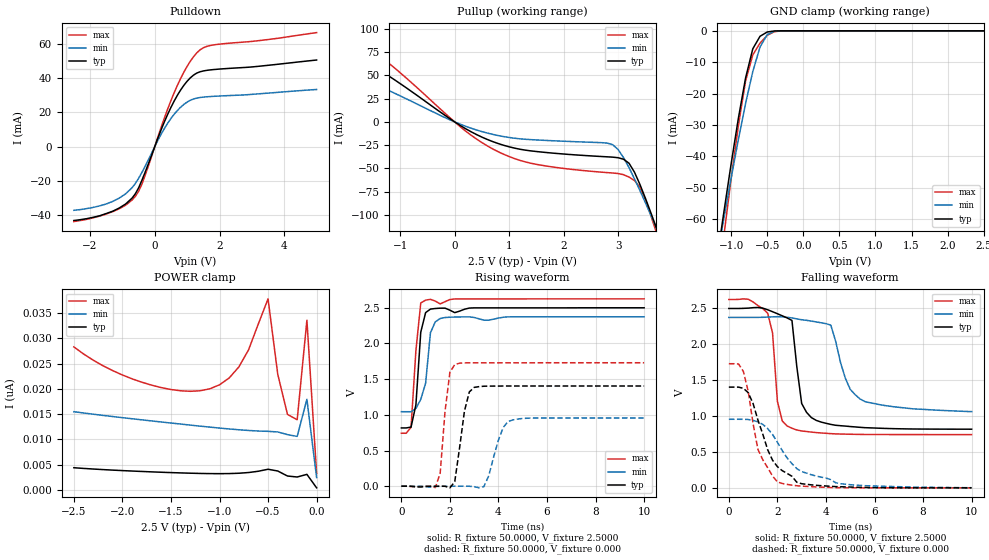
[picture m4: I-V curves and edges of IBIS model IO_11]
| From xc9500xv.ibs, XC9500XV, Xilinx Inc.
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|   Model IO_11
[Model]   IO_11
Model_type   I/O
Polarity   Non-Inverting
Enable   Active-High
Vinl =   0.8000V
Vinh =   2.0000V
Vmeas =   1.2500V
Cref =  35.0000pF
Rref =   1.0000M
Vref =  0.000V
C_comp   1.8820pF   1.2910pF   2.4730pF
[Temperature Range]   25.0000   100.0000   0.000
[Voltage Range]   2.5000V   2.3750V   2.6250V
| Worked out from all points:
|   slope of the pulldown table from 0 to 0.375 V, typ, clamps not added: 21 ohm
|   slope of the pullup table from 0 to 0.375 V, typ, clamps not added: 29.3 ohm
|   GND clamp passes 1 mA (typ) near -0.55 V on its own axis
|   rising waveform, R_fixture 50.0000, V_fixture 2.5000: 20-80 % time 201ps typ, 305ps min, 250ps max; typ from 0.817 V to 2.5 V
|   rising waveform, R_fixture 50.0000, V_fixture 0.000: 20-80 % time 361ps typ, 497ps min, 284ps max; typ from 0 V to 1.4 V
|   falling waveform, R_fixture 50.0000, V_fixture 2.5000: 20-80 % time 383ps typ, 792ps min, 329ps max; typ from 2.5 V to 0.818 V
|   falling waveform, R_fixture 50.0000, V_fixture 0.000: 20-80 % time 1.01ns typ, 1.56ns min, 711ps max; typ from 1.4 V to 0 V
[Pulldown]
| voltage   I(typ)   I(min)   I(max)
-2.5V     -43.3mA    -37.3mA    -43.9mA
-1.9V     -41.4mA    -35.6mA    -41.7mA
-1.3V     -37.85mA   -32.1mA    -38.1mA
-900mV    -33.61mA   -27.65mA   -34.3mA
-600mV    -27.65mA   -21.57mA   -29.14mA
-400mV    -19.86mA   -15.23mA   -22.08mA
200mV     10.04mA    7.385mA    11.51mA
600mV     26.71mA    18.98mA    31.58mA
1V        38.31mA    26.1mA     47.05mA
1.4V      43.85mA    28.77mA    56.7mA
1.8V      45.11mA    29.44mA    59.52mA
5V        50.73mA    33.47mA    66.81mA
[Pullup]
| voltage   I(typ)   I(min)   I(max)
-2.5V     70.1mA     45.22mA    94.12mA
-2.3V     77.89mA    51.6mA     101.4mA
-1.7V     66.38mA    45.58mA    84.64mA
200mV     -7.268mA   -4.674mA   -9.775mA
800mV     -23.24mA   -14.68mA   -32.02mA
1.5V      -31.78mA   -19.37mA   -45.55mA
2.9V      -37.82mA   -24.44mA   -54.84mA
3V        -38.44mA   -29.63mA   -55.39mA
3.2V      -44.33mA   -49.07mA   -59.2mA
3.4V      -67.03mA   -73.55mA   -69.94mA
3.7V      -113.3mA   -113.4mA   -118.3mA
5V        -330.3mA   -295.9mA   -372.6mA
[GND_clamp]
| voltage   I(typ)   I(min)   I(max)
-2.5V     -287.9mA   -252.7mA   -335.8mA
-1.2V     -73.41mA   -72.77mA   -83.79mA
-1.1V     -57.66mA   -59.67mA   -65.18mA
-1V       -42.38mA   -46.9mA    -47.16mA
-900mV    -27.9mA    -34.63mA   -30.27mA
-800mV    -15.03mA   -23.14mA   -16.01mA
-700mV    -5.735mA   -12.98mA   -7.684mA
-600mV    -1.742mA   -5.184mA   -3.919mA
-500mV    -371uA     -1.196mA   -1.434mA
-400mV    -43.13uA   -156.3uA   -255.7uA
-300mV    -2.669uA   -9.838uA   -22.12uA
2.5V      433pA      34.5nA     2.849nA
[POWER_clamp]
| voltage   I(typ)   I(min)   I(max)
-2.5V     4.412nA    15.49nA    28.31nA
-1.8V     3.674nA    13.88nA    21.33nA
-1.4V     3.387nA    13.05nA    19.63nA
-1.1V     3.251nA    12.45nA    20.02nA
-800mV    3.323nA    11.92nA    24.36nA
-700mV    3.464nA    11.78nA    27.76nA
-500mV    4.113nA    11.61nA    37.81nA
-400mV    3.762nA    11.49nA    22.88nA
-300mV    2.773nA    10.96nA    14.96nA
-200mV    2.578nA    10.61nA    13.9nA
-100mV    3.101nA    17.95nA    33.59nA
0V        433.1pA    2.482nA    3.286nA
[Ramp]
| variable   typ   min   max
dV/dt_r   0.8424/0.3291n   0.5735/0.5001n   1.0380/0.2375n
dV/dt_f   1.0095/0.3603n   0.7872/0.6563n   1.1296/0.2494n
R_load = 50.0000
[Rising Waveform]
R_fixture = 50.0000
V_fixture = 2.5000
V_fixture_min = 2.3750
V_fixture_max = 2.6250
L_fixture = 0.000H
C_fixture = 0.000F
| time   V(typ)   V(min)   V(max)
0s        816.6mV    1.044V     742.2mV
400ps     828.4mV    1.044V     824.5mV
600ps     1.14V      1.09V      1.9V
800ps     2.158V     1.216V     2.567V
1ns       2.432V     1.443V     2.607V
1.2ns     2.482V     2.152V     2.618V
1.6ns     2.494V     2.35V      2.554V
2.2ns     2.432V     2.37V      2.623V
3ns       2.499V     2.364V     2.624V
10ns      2.5V       2.374V     2.625V
[Rising Waveform]
R_fixture = 50.0000
V_fixture = 0.000
V_fixture_min = 0.000
V_fixture_max = 0.000
L_fixture = 0.000H
C_fixture = 0.000F
| time   V(typ)   V(min)   V(max)
0s        0V         0V         0V
1.4ns     -272.7uV   -3.587mV   -19.1mV
1.6ns     -41.91uV   -1.078mV   182.6mV
2ns       -22.89mV   -176.5uV   1.597V
2.2ns     63.07mV    -84.99uV   1.704V
2.6ns     1.053V     38.84uV    1.728V
3ns       1.385V     -6.357mV   1.729V
3.4ns     1.401V     -6.205mV   1.729V
4.4ns     1.404V     907.2mV    1.729V
10ns      1.404V     955.9mV    1.73V
[Falling Waveform]
R_fixture = 50.0000
V_fixture = 2.5000
V_fixture_min = 2.3750
V_fixture_max = 2.6250
L_fixture = 0.000H
C_fixture = 0.000F
| time   V(typ)   V(min)   V(max)
0s        2.5V       2.375V     2.625V
1.6ns     2.482V     2.38V      2.434V
2ns       2.427V     2.386V     1.208V
2.4ns     2.369V     2.377V     863.1mV
2.6ns     2.333V     2.369V     830.4mV
3ns       1.176V     2.343V     793.2mV
3.4ns     979.1mV    2.324V     777mV
4.2ns     884.5mV    2.268V     755.7mV
5.4ns     843.7mV    1.24V      744.8mV
10ns      817.5mV    1.063V     742.3mV
[Falling Waveform]
R_fixture = 50.0000
V_fixture = 0.000
V_fixture_min = 0.000
V_fixture_max = 0.000
L_fixture = 0.000H
C_fixture = 0.000F
| time   V(typ)   V(min)   V(max)
0s        1.404V     955.8mV    1.73V
400ps     1.404V     955.8mV    1.727V
600ps     1.387V     955.5mV    1.622V
800ps     1.326V     952.7mV    1.342V
1.2ns     943mV      918.9mV    534.6mV
1.6ns     531.3mV    825.6mV    280.5mV
2ns       295.4mV    635.8mV    82.81mV
2.8ns     78.09mV    267.3mV    29.52mV
4.4ns     17.51mV    71.14mV    3.454mV
10ns      200.5uV    2.204mV    71.67uV
